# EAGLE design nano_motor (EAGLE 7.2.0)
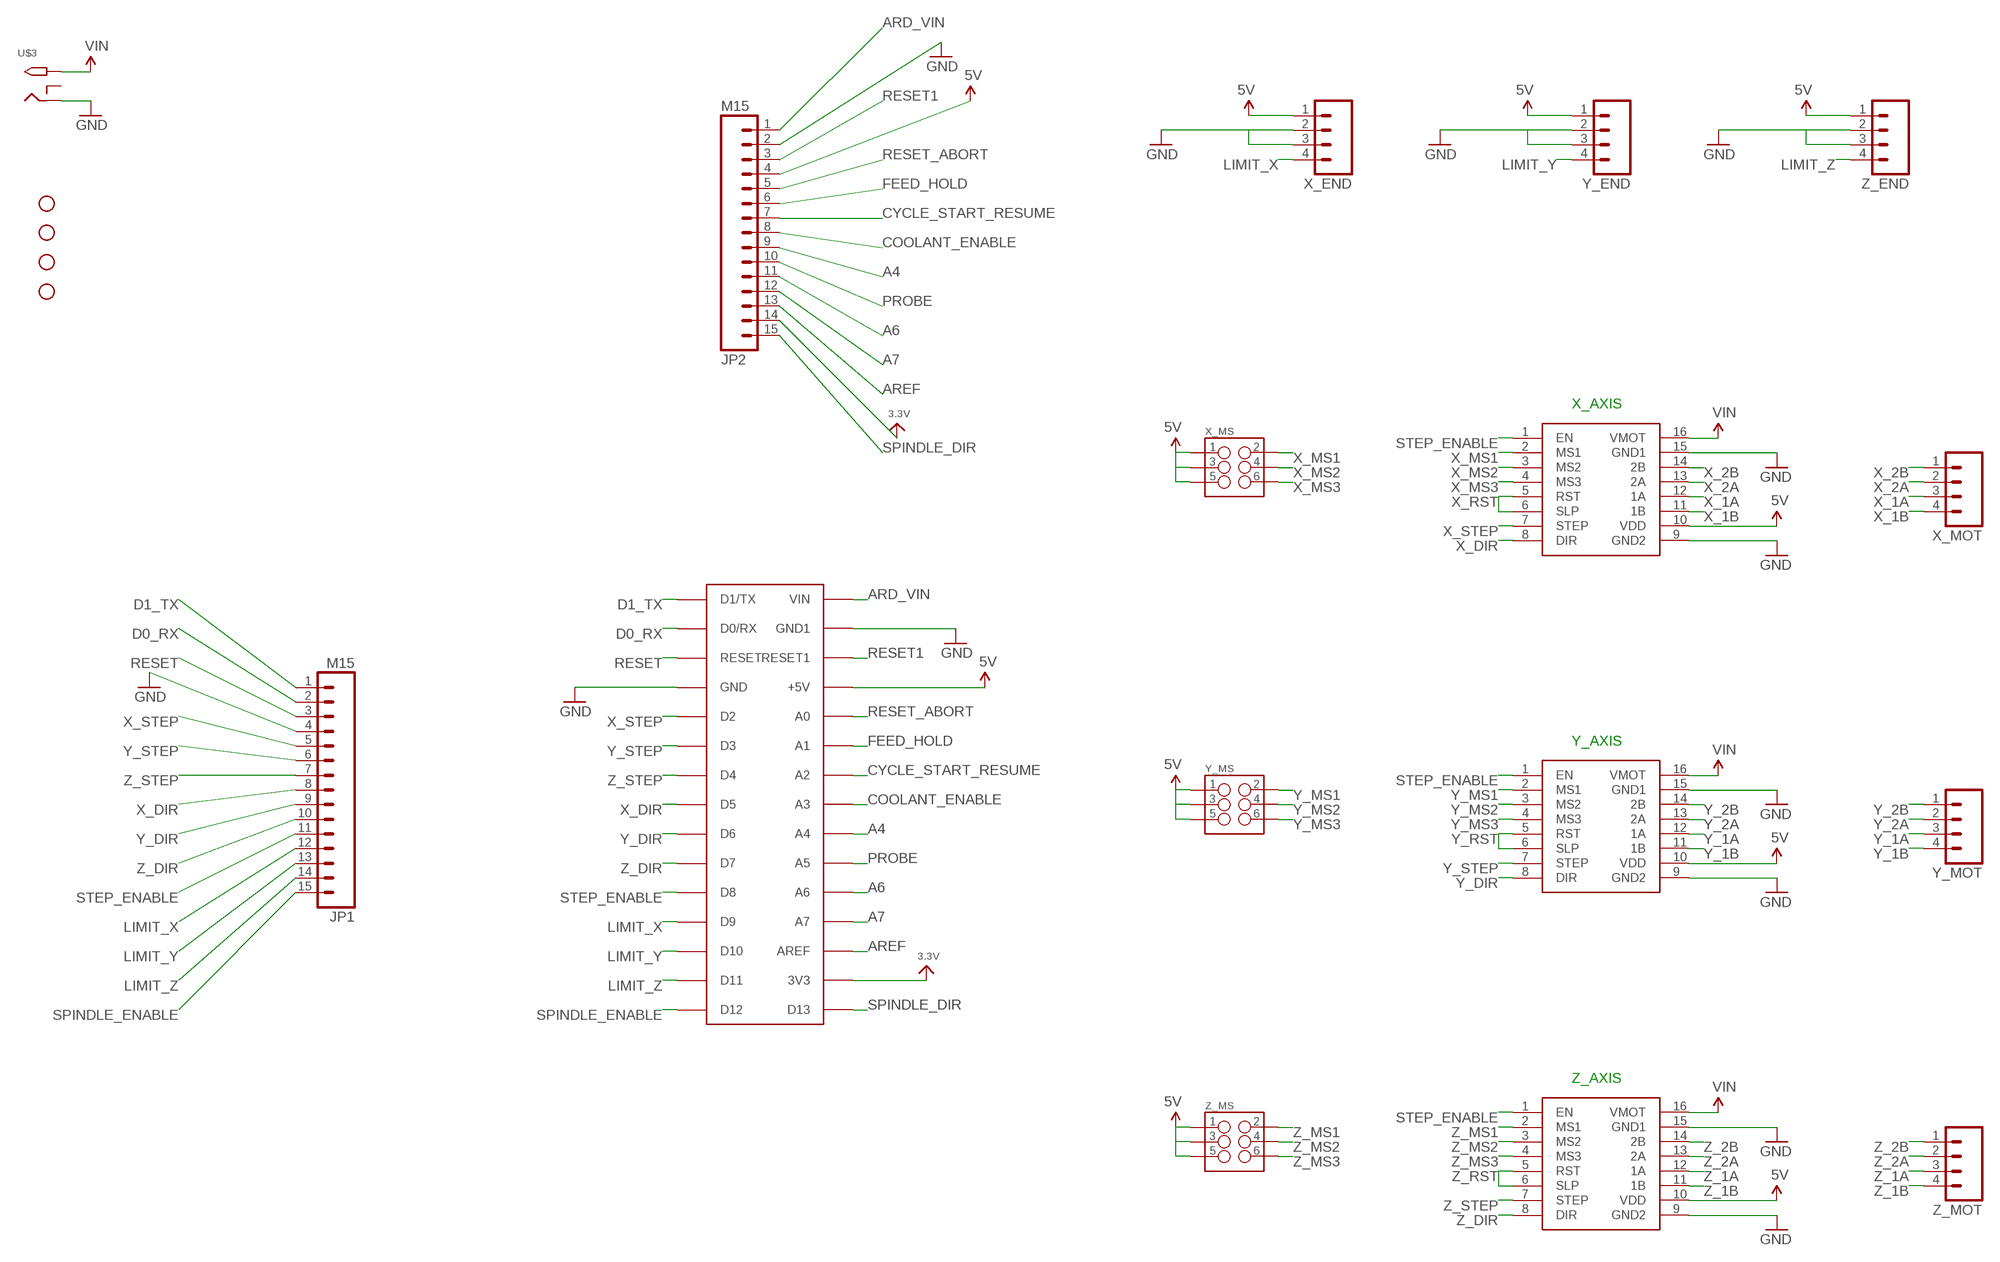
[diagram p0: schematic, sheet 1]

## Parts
JP1  M15  [1X15]
JP2  M15  [1X15]
NANO  ARDUINONANO  [PDIP-32]
STANDOFF1  STAND-OFF  [STAND-OFF]
STANDOFF2  STAND-OFF  [STAND-OFF]
STANDOFF3  STAND-OFF  [STAND-OFF]
STANDOFF4  STAND-OFF  [STAND-OFF]
U$3  2.1MMJACKTHM  [PJ-102A]
X_AXIS  POLOLUESTEPPERDRIVER  [DIL16]
X_END  M04PTH  [1X04]
X_MOT  M04PTH  [1X04]
X_MS  M03X22X3_SILK_SM  [2X3]
Y_AXIS  POLOLUESTEPPERDRIVER  [DIL16]
Y_END  M04PTH  [1X04]
Y_MOT  M04PTH  [1X04]
Y_MS  M03X22X3_SILK_SM  [2X3]
Z_AXIS  POLOLUESTEPPERDRIVER  [DIL16]
Z_END  M04PTH  [1X04]
Z_MOT  M04PTH  [1X04]
Z_MS  M03X22X3_SILK_SM  [2X3]

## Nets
3.3V: JP2.14 NANO.3V3
5V: JP2.4 NANO.+5V X_AXIS.10(VDD) X_END.1 X_MS.1 X_MS.3 X_MS.5 Y_AXIS.10(VDD) Y_END.1 Y_MS.1 Y_MS.3 Y_MS.5 Z_AXIS.10(VDD) Z_END.1 Z_MS.1 Z_MS.3 Z_MS.5
A4: JP2.9 NANO.A4
A6: JP2.11 NANO.A6
A7: JP2.12 NANO.A7
ARD_VIN: JP2.1 NANO.VIN
AREF: JP2.13 NANO.AREF
COOLANT_ENABLE: JP2.8 NANO.A3
CYCLE_START_RESUME: JP2.7 NANO.A2
D0_RX: JP1.2 NANO.D0/RX
D1_TX: JP1.1 NANO.D1/TX
FEED_HOLD: JP2.6 NANO.A1
GND: JP1.4 JP2.2 NANO.GND NANO.GND1 U$3.RING X_AXIS.9(GND2) X_AXIS.15(GND1) X_END.2 X_END.3 Y_AXIS.9(GND2) Y_AXIS.15(GND1) Y_END.2 Y_END.3 Z_AXIS.9(GND2) Z_AXIS.15(GND1) Z_END.2 Z_END.3
LIMIT_X: JP1.12 NANO.D9 X_END.4
LIMIT_Y: JP1.13 NANO.D10 Y_END.4
LIMIT_Z: JP1.14 NANO.D11 Z_END.4
PROBE: JP2.10 NANO.A5
RESET: JP1.3 NANO.RESET
RESET1: JP2.3 NANO.RESET1
RESET_ABORT: JP2.5 NANO.A0
SPINDLE_DIR: JP2.15 NANO.D13
SPINDLE_ENABLE: JP1.15 NANO.D12
STEP_ENABLE: JP1.11 NANO.D8 X_AXIS.1(EN) Y_AXIS.1(EN) Z_AXIS.1(EN)
VIN: U$3.TIP X_AXIS.16(VMOT) Y_AXIS.16(VMOT) Z_AXIS.16(VMOT)
X_1A: X_AXIS.12(1A) X_MOT.3
X_1B: X_AXIS.11(1B) X_MOT.4
X_2A: X_AXIS.13(2A) X_MOT.2
X_2B: X_AXIS.14(2B) X_MOT.1
X_DIR: JP1.8 NANO.D5 X_AXIS.8(DIR)
X_MS1: X_AXIS.2(MS1) X_MS.2
X_MS2: X_AXIS.3(MS2) X_MS.4
X_MS3: X_AXIS.4(MS3) X_MS.6
X_RST: X_AXIS.5(RST) X_AXIS.6(SLP)
X_STEP: JP1.5 NANO.D2 X_AXIS.7(STEP)
Y_1A: Y_AXIS.12(1A) Y_MOT.3
Y_1B: Y_AXIS.11(1B) Y_MOT.4
Y_2A: Y_AXIS.13(2A) Y_MOT.2
Y_2B: Y_AXIS.14(2B) Y_MOT.1
Y_DIR: JP1.9 NANO.D6 Y_AXIS.8(DIR)
Y_MS1: Y_AXIS.2(MS1) Y_MS.2
Y_MS2: Y_AXIS.3(MS2) Y_MS.4
Y_MS3: Y_AXIS.4(MS3) Y_MS.6
Y_RST: Y_AXIS.5(RST) Y_AXIS.6(SLP)
Y_STEP: JP1.6 NANO.D3 Y_AXIS.7(STEP)
Z_1A: Z_AXIS.12(1A) Z_MOT.3
Z_1B: Z_AXIS.11(1B) Z_MOT.4
Z_2A: Z_AXIS.13(2A) Z_MOT.2
Z_2B: Z_AXIS.14(2B) Z_MOT.1
Z_DIR: JP1.10 NANO.D7 Z_AXIS.8(DIR)
Z_MS1: Z_AXIS.2(MS1) Z_MS.2
Z_MS2: Z_AXIS.3(MS2) Z_MS.4
Z_MS3: Z_AXIS.4(MS3) Z_MS.6
Z_RST: Z_AXIS.5(RST) Z_AXIS.6(SLP)
Z_STEP: JP1.7 NANO.D4 Z_AXIS.7(STEP)
Unconnected: U$3.RING_SW

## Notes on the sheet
- X_AXIS
- Y_AXIS
- Z_AXIS

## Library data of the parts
JP1 JP2 = SparkFun-Connectors:M15: Header 15 Standard 15-pin 0.1" header. Use with straight break away headers (SKU : PRT-00116), right angle break away headers (PRT-00553), swiss pins (PRT-00743), machine pins (PRT-00117), and female headers (PRT-00115).
NANO = rocketfarm:ARDUINONANO
STANDOFF1-STANDOFF4 = SparkFun-Electromechanical:STAND-OFF: #4 Stand Off
U$3 = adafruit:2.1MMJACK: 2.1mm x 5.5mm THM DC jack with internal switch. Digikey part #PJ-102A, 4UCON part #05537 2.1mm x 5.5mm SMT DC jack with internal switch. Digikey part #PJ-002A-SMT, 4UCON part #03267 By microbuilder.eu & adafruit.com
X_AXIS Y_AXIS Z_AXIS = reprap:POLOLUESTEPPERDRIVER: Pololu stepper driver based on the A4983.
X_END X_MOT Y_END Y_MOT Z_END Z_MOT = SparkFun-Connectors:M04: Header 4 Standard 4-pin 0.1" header. Use with straight break away headers (SKU : PRT-00116), right angle break away headers (PRT-00553), swiss pins (PRT-00743), machine pins (PRT-00117), and female headers (PRT-00115). Molex polarized connector foot print use with SKU : PRT-08231 with associated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
X_MS Y_MS Z_MS = SparkFun-Connectors:M03X2: 2x3 .1" header. Shrouded, with keying- CONN-10681 SMT- CONN-11415 Pogo pins- HW-11044

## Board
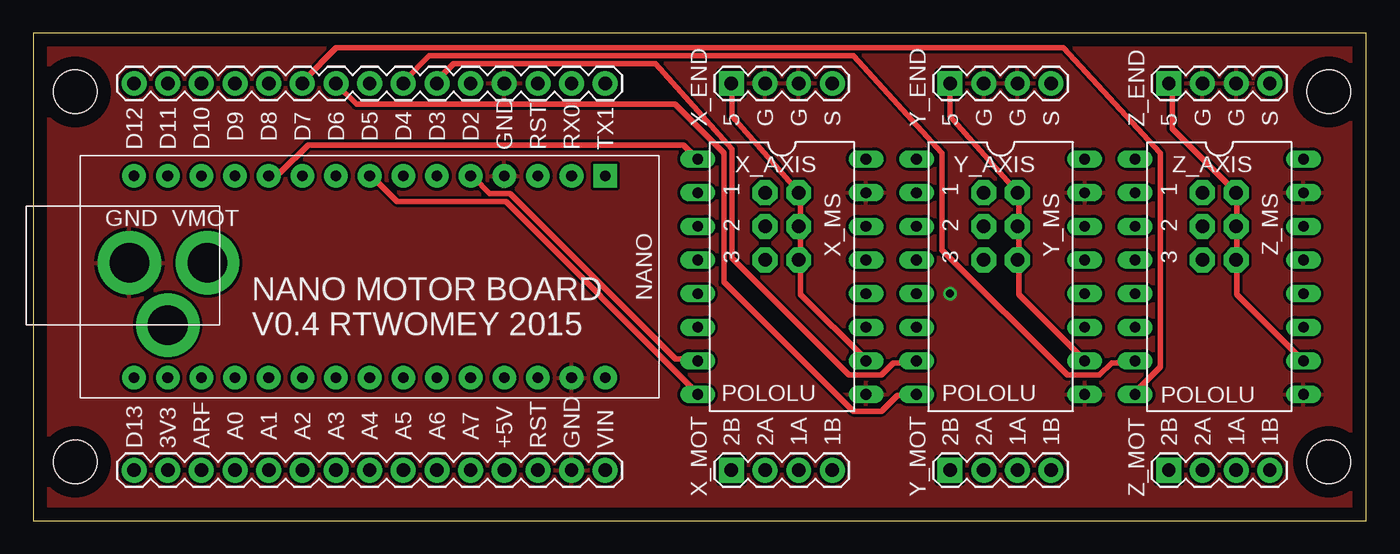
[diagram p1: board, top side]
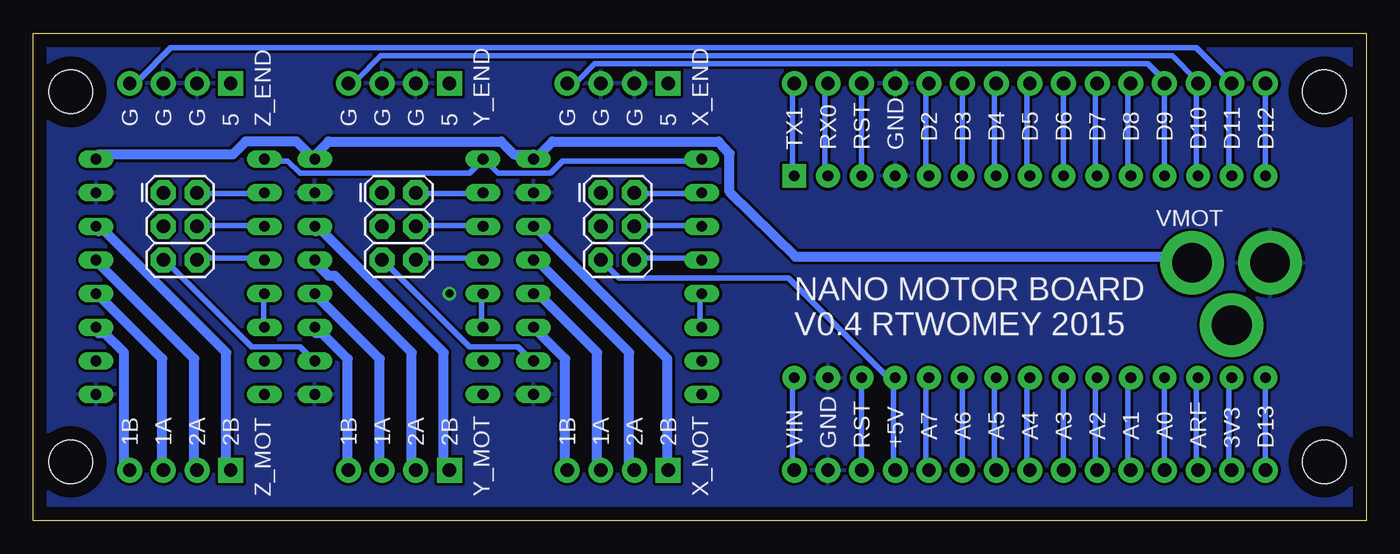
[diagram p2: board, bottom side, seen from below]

Size 100.64 x 36.82 mm. Coordinates in mm from the lower left corner, seen from the top.
Outline: 0,0 100.64,0 100.64,36.82 0,36.82 0,0
Copper layers (1*16): Top 0.035mm / dielectric 1.5mm / Bottom 0.035mm
Design rules "default *": minimum track width 16mil, minimum drill 24mil, track to track 8mil, track to pad 8mil, pad to pad 8mil, via to via 8mil, smd to smd 8mil, copper to edge 40mil, drill to drill 8mil, minimum pad ring 10mil, minimum via ring 8mil, stop-mask expansion 4mil, vias tented up to drill 0mil, thermal gap 10mil

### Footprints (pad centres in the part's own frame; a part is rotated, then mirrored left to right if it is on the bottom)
1X15 = drill 1.016 pad 1.88: 1 0,0; 2 2.54,0; 3 5.08,0; 4 7.62,0; 5 10.16,0; 6 12.7,0; 7 15.24,0; 8 17.78,0; 9 20.32,0; 10 22.86,0; 11 25.4,0; 12 27.94,0; 13 30.48,0; 14 33.02,0; 15 35.56,0
PDIP-32 = drill 0.8 pad 1.778: 3V3 15.24,-35.56; +5V 15.24,-10.16; A0 15.24,-12.7; A1 15.24,-15.24; A2 15.24,-17.78; A3 15.24,-20.32; A4 15.24,-22.86; A5 15.24,-25.4; A6 15.24,-27.94; A7 15.24,-30.48; AREF 15.24,-33.02; D0/RX 0,-5.08; D2 0,-12.7; D3 0,-15.24; D4 0,-17.78; D5 0,-20.32; D6 0,-22.86; D7 0,-25.4; D8 0,-27.94; D9 0,-30.48; D10 0,-33.02; D11 0,-35.56; D12 0,-38.1; D13 15.24,-38.1; GND 0,-10.16; GND1 15.24,-5.08; RESET 0,-7.62; RESET1 15.24,-7.62; VIN 15.24,-2.54 | drill 0.8 pad 1.778 square: D1/TX 0,-2.54
STAND-OFF = hole 3.302: 0,0
PJ-102A = drill 3 pad 4.8: RING 0.1,-3.39; RING_SW -4.6,-6.29; TIP 0.1,-9.29
DIL16 = drill 0.813 long: 1 -6.35,8.89; 2 -6.35,6.35; 3 -6.35,3.81; 4 -6.35,1.27; 5 -6.35,-1.27; 6 -6.35,-3.81; 7 -6.35,-6.35; 8 -6.35,-8.89; 9 6.35,-8.89; 10 6.35,-6.35; 11 6.35,-3.81; 12 6.35,-1.27; 13 6.35,1.27; 14 6.35,3.81; 15 6.35,6.35; 16 6.35,8.89
1X04 = drill 1.016 pad 1.88 square: 1 0,0 | drill 1.016 pad 1.88: 2 2.54,0; 3 5.08,0; 4 7.62,0
2X3 = drill 1.016 pad 1.88 octagon: 1 0,0; 2 0,2.54; 3 2.54,0; 4 2.54,2.54; 5 5.08,0; 6 5.08,2.54

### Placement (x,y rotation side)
JP1  43.18,33.02 180 top
JP2  43.18,3.81 180 top
NANO  45.72,26.04 270 top
STANDOFF1  3.17,4.45 0 top
STANDOFF2  97.79,4.45 0 top
STANDOFF3  97.79,32.38 0 top
STANDOFF4  3.17,32.38 0 top
U$3  3.87,19.37 90 top
X_AXIS  56.52,18.41 0 top
X_END  52.7,33.02 0 top
X_MOT  52.7,3.81 0 top
X_MS  57.78,24.77 270 bottom
Y_AXIS  73.03,18.41 0 top
Y_END  69.22,33.02 0 top
Y_MOT  69.22,3.81 0 top
Y_MS  74.3,24.77 270 bottom
Z_AXIS  89.53,18.41 0 top
Z_END  85.72,33.02 0 top
Z_MOT  85.72,3.81 0 top
Z_MS  90.81,24.77 270 bottom

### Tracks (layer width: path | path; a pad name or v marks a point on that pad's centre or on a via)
3.3V
  Bottom 0.406: NANO.3V3 10.39,10.69 10.39,3.96 JP2.14
5V
  Top 0.406: Z_MS.5 90.86,19.84 90.86,21.97 Z_MS.3 90.86,22.28 90.86,24.71 Z_MS.1 85.98,29.59 85.98,32.97 Z_END.1 | Y_MS.5 74.4,19.84 74.4,21.97 Y_MS.3 74.4,22.28 74.4,24.71 Y_MS.1 74.09,25.02 69.22,30.53 Y_END.1 | Z_AXIS.10 90.86,17.09 90.86,19.53 Z_MS.5 | Y_MS.5 74.4,19.53 74.4,17.09 79.27,12.22 Y_AXIS.10 79.58,12.22 | X_END.1 52.76,32.97 52.76,30.53 57.63,25.02 X_MS.1 57.94,24.71 57.94,22.28 X_MS.3 57.94,21.97 57.94,19.84 X_MS.5 57.94,19.53 57.94,17.09 62.81,12.22 X_AXIS.10 63.12,12.22 | 74.09,19.53 Y_MS.5 | 90.55,19.53 Z_MS.5
  Bottom 0.406: JP2.4 35.69,3.96 35.69,10.69 NANO.+5V 35.69,11 36.3,11 43.61,18.31 56.41,18.31 X_MS.5 | X_AXIS.10 63.12,12.22 64.03,13.13 67.69,13.13 74.09,19.53 Y_MS.5 | Y_AXIS.10 79.58,12.22 80.49,13.13 84.15,13.13 90.55,19.53 Z_MS.5
A4
  Bottom 0.406: NANO.A4 22.89,10.69 22.89,3.96 JP2.9
A6
  Bottom 0.406: NANO.A6 18.01,10.69 18.01,3.96 JP2.11
A7
  Bottom 0.406: NANO.A7 15.27,10.69 15.27,3.96 JP2.12
ARD_VIN
  Bottom 0.406: NANO.VIN 43.31,10.69 43.31,3.96 JP2.1
AREF
  Bottom 0.406: NANO.AREF 12.83,10.69 12.83,3.96 JP2.13
COOLANT_ENABLE
  Bottom 0.406: NANO.A3 25.63,10.69 25.63,3.96 JP2.8
CYCLE_START_RESUME
  Bottom 0.406: NANO.A2 28.07,10.69 28.07,3.96 JP2.7
D0_RX
  Bottom 0.406: NANO.D0/RX 40.87,26.24 40.87,32.97 JP1.2
D1_TX
  Bottom 0.406: NANO.D1/TX 43.31,26.24 43.31,32.97 JP1.1
FEED_HOLD
  Bottom 0.406: NANO.A1 30.5,10.69 30.5,3.96 JP2.6
GND  (via drill 0.6)
  other vias: 69.22,17.14
  pour Top: 0,0 0,37.47 100.97,37.47 100.97,0
  pour Bottom: 0,0 0,36.83 100.97,36.83 100.97,0
LIMIT_X
  Bottom 0.406: NANO.D9 15.27,26.24 15.27,32.97 JP1.12 15.27,33.27 16.48,34.49 58.24,34.49 59.46,33.27 60.07,33.27 X_END.4
LIMIT_Y
  Bottom 0.406: NANO.D10 12.83,26.24 12.83,32.97 JP1.13 12.83,33.27 14.66,35.1 74.4,35.1 76.22,33.27 76.83,33.27 Y_END.4
LIMIT_Z
  Bottom 0.406: NANO.D11 10.39,26.24 10.39,32.97 JP1.14 10.39,33.27 12.83,35.71 90.25,35.71 92.69,33.27 93.29,33.27 Z_END.4
PROBE
  Bottom 0.406: NANO.A5 20.45,10.69 20.45,3.96 JP2.10
RESET
  Bottom 0.406: NANO.RESET 38.12,26.24 38.12,32.97 JP1.3
RESET1
  Bottom 0.406: NANO.RESET1 38.12,10.69 38.12,3.96 JP2.3
RESET_ABORT
  Bottom 0.406: NANO.A0 33.25,10.69 33.25,3.96 JP2.5
SPINDLE_DIR
  Bottom 0.406: NANO.D13 7.64,10.69 7.64,3.96 JP2.15
SPINDLE_ENABLE
  Bottom 0.406: NANO.D12 7.64,26.24 7.64,32.97 JP1.15
STEP_ENABLE
  Top 0.406: X_AXIS.1 49.1,28.37 20.75,28.37 18.62,26.24 18.01,26.24 NANO.D8
  Bottom 0.406: JP1.11 18.01,32.97 18.01,26.24 NANO.D8 | X_AXIS.1 50.32,27.15 60.68,27.15 61.59,26.24 65.56,26.24 66.47,27.15 Y_AXIS.1 66.78,27.15 67.69,26.24 80.49,26.24 81.41,27.15 82.93,27.15 Z_AXIS.1
VIN
  Bottom 0.762: Z_AXIS.16 95.71,27.66 85.57,27.66 84.61,28.63 80.75,28.63 79.78,27.66 Y_AXIS.16 79.3,27.66 78.33,28.63 65.3,28.63 64.34,27.66 62.89,27.66 X_AXIS.16 62.41,27.66 61.44,28.63 48.9,28.63 48.06,27.72 48.06,24.83 43.1,19.94 13.18,19.94 U$3.TIP
X_1A
  Bottom 0.762: X_AXIS.12 62.41,17.04 58.06,12.7 58.06,3.86 X_MOT.3
X_1B
  Bottom 0.762: X_AXIS.11 60.48,12.22 60.48,3.86 X_MOT.4
X_2A
  Bottom 0.762: X_AXIS.13 62.41,19.46 55.65,12.7 55.65,3.86 X_MOT.2
X_2B
  Bottom 0.762: X_AXIS.14 62.41,21.87 52.76,12.22 52.76,3.86 X_MOT.1
X_DIR
  Top 0.406: X_AXIS.8 50.01,9.78 35.69,24.11 27.46,24.11 25.63,25.93 NANO.D5
  Bottom 0.406: JP1.8 25.63,32.97 25.63,26.24 NANO.D5
X_MS1
  Bottom 0.406: X_AXIS.2 50.32,24.71 55.19,24.71 X_MS.2
X_MS2
  Bottom 0.406: X_AXIS.3 50.32,22.28 55.19,22.28 X_MS.4
X_MS3
  Bottom 0.406: X_AXIS.4 50.32,19.84 55.19,19.84 X_MS.6
X_RST
  Bottom 0.406: X_AXIS.6 50.32,14.66 50.32,17.09 X_AXIS.5
X_STEP
  Top 0.406: X_AXIS.7 50.01,12.22 48.49,12.22 35.99,24.71 34.47,24.71 33.25,25.93 NANO.D2
  Bottom 0.406: JP1.5 33.25,32.97 33.25,26.24 NANO.D2
Y_1A
  Bottom 0.762: Y_AXIS.12 79.3,17.04 74.47,12.22 74.47,3.86 Y_MOT.3
Y_1B
  Bottom 0.762: Y_AXIS.11 79.3,14.15 78.82,14.15 76.89,12.22 76.89,3.86 Y_MOT.4
Y_2A
  Bottom 0.762: Y_AXIS.13 79.3,19.46 78.33,18.49 77.85,18.49 72.06,12.7 72.06,3.86 Y_MOT.2
Y_2B
  Bottom 0.406: 69.65,3.96 69.22,3.96 Y_MOT.1
  Bottom 0.762: 69.65,3.86 69.65,3.96 69.65,12.7 78.82,21.87 79.3,21.87 Y_AXIS.14
Y_DIR
  Top 0.406: Y_AXIS.8 66.47,9.47 65.25,9.47 64.03,8.26 61.9,8.26 52.15,18.01 52.15,27.76 48.46,31.45 24.41,31.45 22.89,32.97 JP1.9
  Bottom 0.406: NANO.D6 22.89,26.24 22.89,32.97 JP1.9
Y_MS1
  Bottom 0.406: Y_AXIS.2 66.78,24.71 71.65,24.71 Y_MS.2
Y_MS2
  Bottom 0.406: Y_AXIS.3 66.78,22.28 71.65,22.28 Y_MS.4
Y_MS3
  Bottom 0.406: Y_AXIS.4 66.78,19.84 71.65,19.84 Y_MS.6
Y_RST
  Bottom 0.406: Y_AXIS.6 66.78,14.66 66.78,17.09 Y_AXIS.5
Y_STEP
  Top 0.406: Y_AXIS.7 66.47,11.91 64.95,11.91 64.03,11 61.59,11 52.76,19.84 52.76,28.07 46.97,34.49 31.73,34.49 30.5,33.27 JP1.6
  Bottom 0.406: NANO.D3 30.5,26.24 30.5,32.97 JP1.6
Z_1A
  Bottom 0.762: Z_AXIS.12 95.71,17.04 90.88,12.22 90.88,3.86 Z_MOT.3
Z_1B
  Bottom 0.762: Z_AXIS.11 95.71,14.15 95.22,14.15 93.78,12.7 93.78,3.86 Z_MOT.4
Z_2A
  Bottom 0.762: Z_AXIS.13 95.71,19.46 88.47,12.22 88.47,3.86 Z_MOT.2
Z_2B
  Bottom 0.762: Z_MOT.1 86.06,3.86 86.06,12.7 95.22,21.87 95.71,21.87 Z_AXIS.14
Z_DIR
  Top 0.406: Z_AXIS.8 83.24,9.78 85.06,11.61 85.06,27.76 77.75,35.71 22.89,35.71 20.45,33.27 JP1.10 20.45,32.97
  Bottom 0.406: NANO.D7 20.45,26.24 20.45,32.97 JP1.10
Z_MS1
  Bottom 0.406: Z_AXIS.2 83.24,24.71 88.11,24.71 Z_MS.2
Z_MS2
  Bottom 0.406: Z_AXIS.3 83.24,22.28 88.11,22.28 Z_MS.4
Z_MS3
  Bottom 0.406: Z_AXIS.4 83.24,19.84 88.11,19.84 Z_MS.6
Z_RST
  Bottom 0.406: Z_AXIS.6 83.24,14.66 83.24,17.09 Z_AXIS.5
Z_STEP
  Top 0.406: Z_AXIS.7 82.93,11.91 81.41,11.91 80.49,11 78.05,11 68.61,20.45 68.61,27.76 61.9,35.1 29.9,35.1 28.07,33.27 JP1.7 28.07,32.97
  Bottom 0.406: NANO.D4 28.07,26.24 28.07,32.97 JP1.7

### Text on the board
tNames: 5 | G | G | S | 5 | G | G | S | 5 | G | G | S | D9 | D8 | D7 | D6 | D5 | D4 | D3 | D2 | D12 | D11 | D10 | GND | RST | RX0 | TX1 | 1 | 1 | 1 | GND | VMOT | 2 | 2 | 2 | 3 | 3 | 3 | NANO MOTOR BOARD / V0.4 RTWOMEY 2015 | POLOLU | POLOLU | POLOLU | A0 | A1 | A2 | A3 | A4 | A5 | A6 | A7 | 2B | 2A | 1A | 1B | 2B | 2A | 1A | 1B | 2B | 2A | 1A | 1B | D13 | 3V3 | ARF | +5V | RST | GND | VIN
bNames: X_END | 5 | G | G | G | Y_END | 5 | G | G | G | Z_END | 5 | G | G | G | D9 | D8 | D7 | D6 | D5 | D4 | D3 | D2 | D12 | D11 | D10 | GND | RST | RX0 | TX1 | VMOT | NANO MOTOR BOARD / V0.4 RTWOMEY 2015 | A0 | A1 | A2 | A3 | A4 | A5 | A6 | A7 | 2B | 2A | 1A | 1B | 2B | 2A | 1A | 1B | 2B | 2A | 1A | 1B | D13 | 3V3 | ARF | +5V | RST | GND | VIN | X_MOT | Y_MOT | Z_MOT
